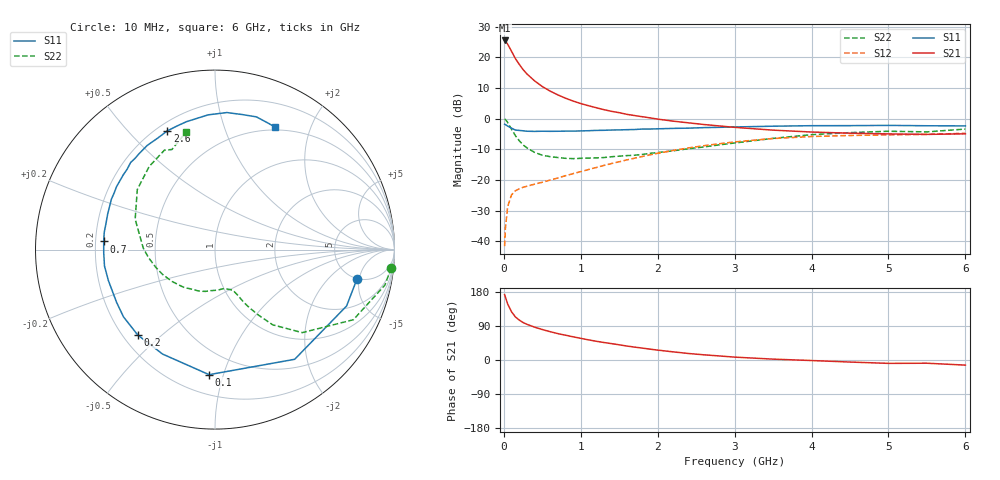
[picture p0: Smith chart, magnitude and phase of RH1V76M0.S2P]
! SIEMENS Small Signal Semiconductors
! BFR106
! Si NPN RF Bipolar Junction Transistor in SOT23
! VCE = 1.75 V  IC = 6 mA
! Common Emitter S-Parameters:  August  1996
# GHz  S  MA  R  50
!  f  S11  S21  S12  S22
! GHz  MAG  ANG  MAG  ANG  MAG  ANG  MAG  ANG
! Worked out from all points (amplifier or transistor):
!   36 points, 10 MHz to 6 GHz, reference 50 ohm
!   highest |S21| = 25.5 dB at 10 MHz (marker M1)
!   |S21| within 3 dB of that: start of sweep to 88.4 MHz
!   unconditionally stable (mu >= 1): 568.7 MHz to 2.36 GHz; 4.211 GHz to end of sweep
!   at 250 MHz: K = 0.56, MSG = 19.2 dB, |S12| = -22.4 dB
!   at 1.4 GHz: K = 1.15, MAG = 6.2 dB, |S12| = -14.7 dB
!   at 6 GHz: K = 1.03, MAG = -1.1 dB, |S12| = -4.8 dB
!   S11 on the Smith chart (normalised r, x): 10 MHz: 4.93, -4.65; 100 MHz: 0.33, -0.90; 200 MHz: 0.26, -0.42; 700 MHz: 0.23, +0.03; 2.6 GHz: 0.24, +0.65; 6 GHz: 0.47, +1.51
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0.01  0.8079 -11.7  18.82 172.4  0.0083 85.8  0.9869 -5.9
0.02  0.7976 -23.2  18.46 166.2  0.0162 80.4  0.9674 -11.8
0.05  0.7554 -54.0  16.31 147.7  0.0369 63.8  0.8641 -26.9
0.1  0.6976 -92.7  12.54 127.3  0.057 49.2  0.6708 -43.6
0.15  0.6512 -116.7  9.564 113.7  0.0665 41.1  0.5282 -52.5
0.2  0.6415 -132.2  7.693 105.4  0.0716 38.2  0.4366 -56.5
0.25  0.6327 -143.7  6.311 98.9  0.0757 37.1  0.3712 -59.6
0.3  0.6222 -151.7  5.351 94.2  0.0789 37.5  0.3336 -61.4
0.4  0.6185 -163.8  4.123 86.7  0.0853 39.2  0.281 -63.7
0.5  0.6225 -171.6  3.334 80.4  0.0916 41.7  0.2526 -65.7
0.6  0.6202 -178.6  2.816 74.8  0.0992 44.4  0.2396 -68.6
0.7  0.6218 175.8  2.444 69.7  0.1073 47.1  0.2318 -72.1
0.9  0.6245 166.6  1.935 61.2  0.1264 51.3  0.2223 -79.2
1.1  0.6343 158.0  1.623 53.2  0.1475 53.8  0.2267 -88.7
1.3  0.6444 150.7  1.4 46.2  0.1722 55.2  0.2315 -98.0
1.6  0.6595 140.7  1.173 36.8  0.2121 55.5  0.2491 -113.1
2.2  0.6924 123.1  0.909 21.5  0.302 50.3  0.2984 -143.6
2.6  0.7127 111.9  0.801 13.7  0.3614 44.5  0.3447 -163.4
3.5  0.7517 92.9  0.648 2.3  0.4732 28.5  0.4757 159.2
4.5  0.7676 78.5  0.578 -5.4  0.5305 11.3  0.5906 128.4
5.5  0.7643 67.2  0.553 -8.5  0.5523 0.9  0.6071 113.3
6  0.7599 63.7  0.564 -13.5  0.5758 -6.4  0.6755 103.7
